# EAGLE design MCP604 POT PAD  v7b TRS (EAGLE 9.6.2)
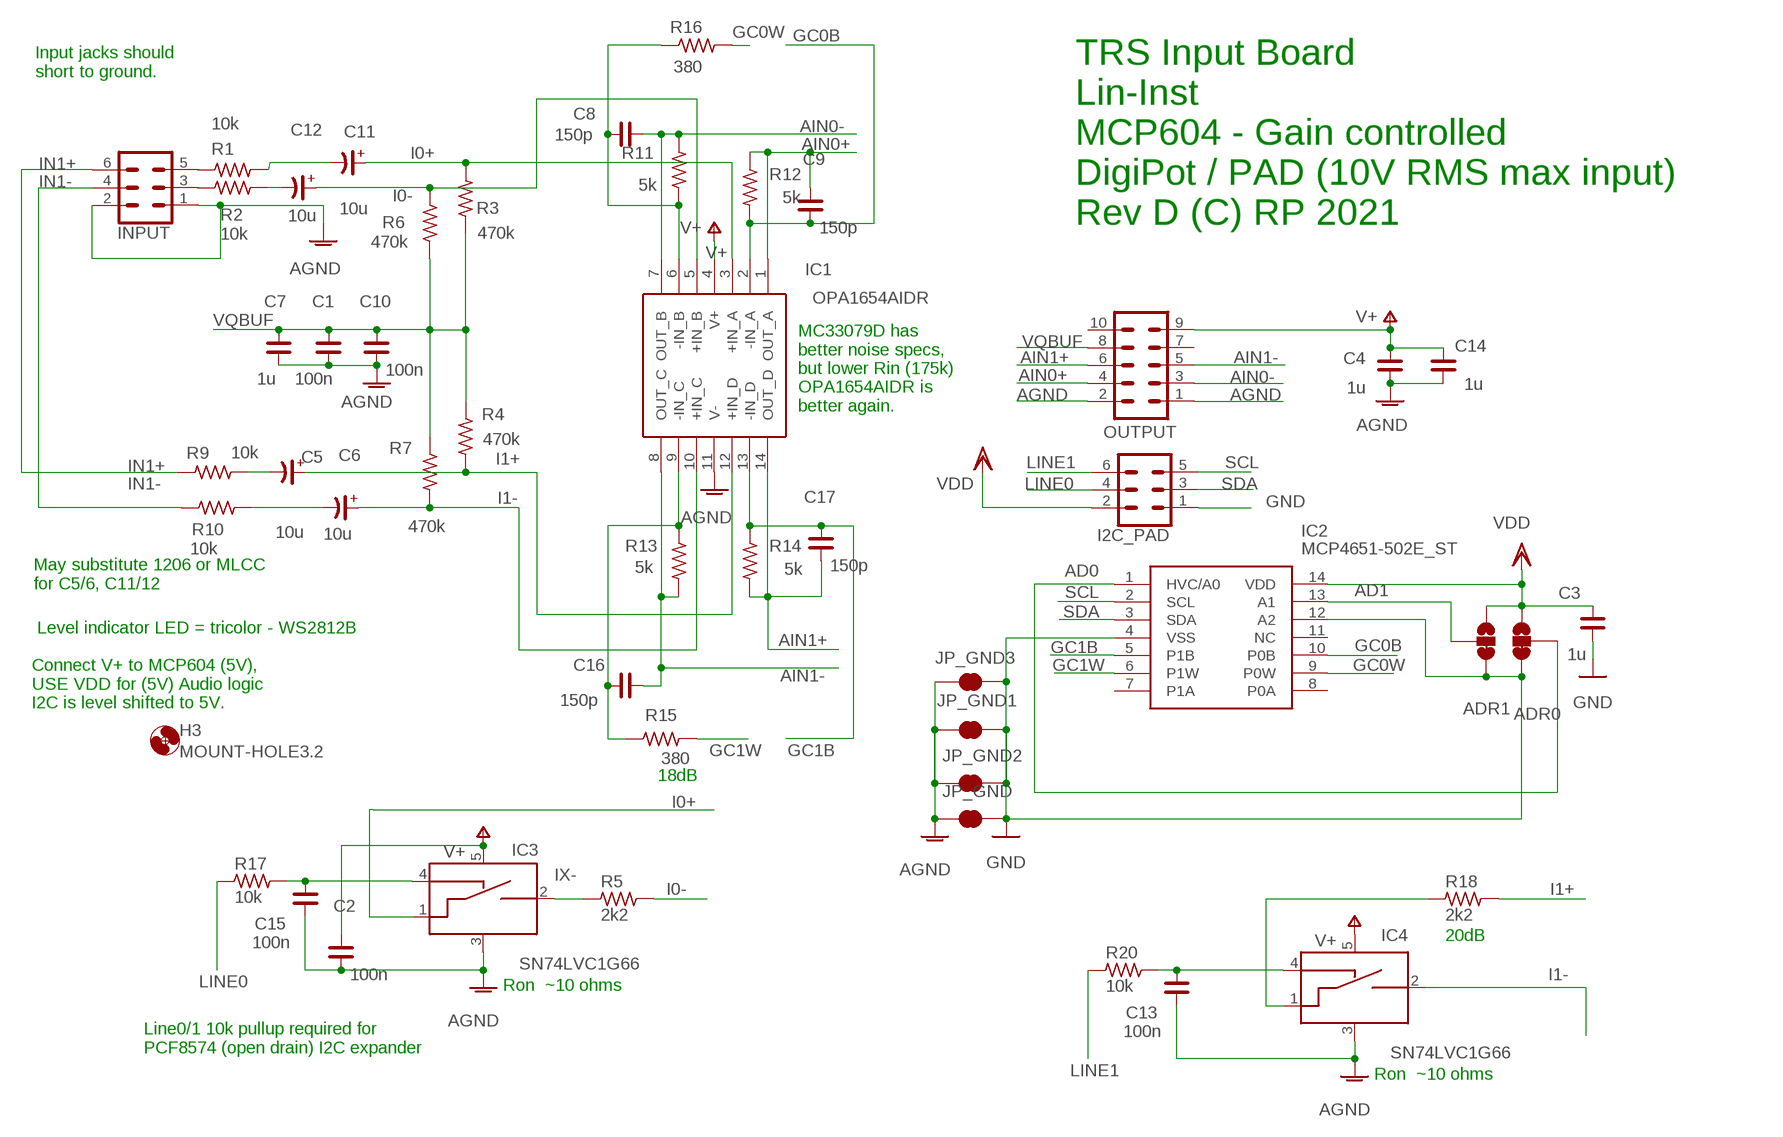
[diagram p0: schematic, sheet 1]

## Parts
ADR0  JUMPER-SMT_3_1-NC_TRACE_SILK  [SMT-JUMPER_3_1-NC_TRACE_SILK]
ADR1  JUMPER-SMT_3_1-NC_TRACE_SILK  [SMT-JUMPER_3_1-NC_TRACE_SILK]
C1  100n  C_0805  [C0805]
C2  100n  C_0805  [C0805]
C3  1u  C_0805  [C0805]
C4  1u  C_0805  [C0805]
C5  10u  CP_SV-B  [CSV-B]
C6  10u  CP_SV-B  [CSV-B]
C7  1u  C_0805  [C0805]
C8  150p  C_0805  [C0805]
C9  150p  C_0805  [C0805]
C10  100n  C_0805  [C0805]
C11  10u  CP_SV-B  [CSV-B]
C12  10u  CP_SV-B  [CSV-B]
C13  100n  C_0805  [C0805]
C14  1u  C_0805  [C0805]
C15  100n  C_0805  [C0805]
C16  150p  C_0805  [C0805]
C17  150p  C_0805  [C0805]
H3  MOUNT-HOLE3.2  [3,2]
I2C_PAD  CONN_03X2SHROUD  [2X3-SHROUDED]
IC1  OPA1654AIDR  [SOIC127P600X175-14N]
IC2  MCP4651-502E_ST  [SOP65P640X120-14N]
IC3  SN74LVC1G66  74LVC1G66  [SOT23-5]
IC4  SN74LVC1G66  74LVC1G66  [SOT23-5]
INPUT  CONN_03X2SHROUD  [2X3-SHROUDED]
JP_GND  JUMPER-SMT_2_NC_TRACE_NO-SILK  [SMT-JUMPER_2_NC_TRACE_NO-SILK]
JP_GND1  JUMPER-SMT_2_NC_TRACE_NO-SILK  [SMT-JUMPER_2_NC_TRACE_NO-SILK]
JP_GND2  JUMPER-SMT_2_NC_TRACE_NO-SILK  [SMT-JUMPER_2_NC_TRACE_NO-SILK]
JP_GND3  JUMPER-SMT_2_NC_TRACE_NO-SILK  [SMT-JUMPER_2_NC_TRACE_NO-SILK]
OUTPUT  CONN_05X2SHD_LOCK  [2X5-SHROUDED_LOCK]
R1  10k  R_0805  [R0805]
R2  10k  R_0805  [R0805]
R3  470k  R_0805  [R0805]
R4  470k  R_0805  [R0805]
R5  2k2  R_0805  [R0805]
R6  470k  R_0805  [R0805]
R7  470k  R_0805  [R0805]
R9  10k  R_0805  [R0805]
R10  10k  R_0805  [R0805]
R11  5k  R_0805  [R0805]
R12  5k  R_0805  [R0805]
R13  5k  R_0805  [R0805]
R14  5k  R_0805  [R0805]
R15  380  R_0805  [R0805]
R16  380  R_0805  [R0805]
R17  10k  R_0805  [R0805]
R18  2k2  R_0805  [R0805]
R20  10k  R_0805  [R0805]

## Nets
AD0: ADR0.2 IC2.1(HVC/A0)
AD1: ADR1.2 IC2.13(A1)
AGND: C1.1 C2.1 C4.1 C7.1 C10.1 C13.1 C14.1 C15.1 IC1.11(V-) IC3.3(VSS) IC4.3(VSS) INPUT.1 INPUT.2 JP_GND1.1 JP_GND2.1 JP_GND3.1 JP_GND.1 OUTPUT.1 OUTPUT.2
AIN0+: C9.2 IC1.1(OUT_A) OUTPUT.4 R12.2
AIN0-: C8.1 IC1.7(OUT_B) OUTPUT.3 R11.2
AIN1+: C17.1 IC1.14(OUT_D) OUTPUT.6 R14.1
AIN1-: C16.1 IC1.8(OUT_C) OUTPUT.5 R13.1
GC0B: C9.1 IC1.2(-IN_A) IC2.10(P0B) R12.1
GC0W: IC2.9(P0W) R16.1
GC1B: C17.2 IC1.13(-IN_D) IC2.5(P1B) R14.2
GC1W: IC2.6(P1W) R15.1
GND: ADR0.3 ADR1.3 C3.1 I2C_PAD.1 IC2.4(VSS) IC2.12(A2) JP_GND1.2 JP_GND2.2 JP_GND3.2 JP_GND.2
I0+: C11.+ IC1.3(+IN_A) IC3.1(A_IN) R3.2
I0-: C12.+ IC1.5(+IN_B) R5.2 R6.2
I1+: C5.+ IC1.12(+IN_D) R4.1 R18.2
I1+X: IC4.1(A_IN) R18.1
I1-: C6.+ IC1.10(+IN_C) IC4.2(A_OUT) R7.1
IN1+: INPUT.6 R9.1
IN1-: INPUT.4 R10.1
IX-: IC3.2(A_OUT) R5.1
LINE0: I2C_PAD.4 R17.1
LINE1: I2C_PAD.6 R20.1
N$2: C12.- R2.2
N$4: C13.2 IC4.4(CTRL_IN) R20.2
N$5: C8.2 IC1.6(-IN_B) R11.1 R16.2
N$6: INPUT.5 R1.1
N$7: C16.2 IC1.9(-IN_C) R13.2 R15.2
N$8: INPUT.3 R2.1
N$9: C11.- R1.2
N$15: C15.2 IC3.4(CTRL_IN) R17.2
N$18: C5.- R9.2
N$19: C6.- R10.2
SCL: I2C_PAD.5 IC2.2(SCL)
SDA: I2C_PAD.3 IC2.3(SDA)
V+: C2.2 C4.2 C14.2 IC1.4(V+) IC3.5(VCC) IC4.5(VCC) OUTPUT.9
VDD: ADR0.1 ADR1.1 C3.2 I2C_PAD.2 IC2.14(VDD)
VQBUF: C1.2 C7.2 C10.2 OUTPUT.8 R3.1 R4.2 R6.1 R7.2
Unconnected: IC2.7(P1A) IC2.8(P0A) IC2.11(NC) OUTPUT.7 OUTPUT.10

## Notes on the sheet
- Input jacks should 
  short to ground.
- TRS Input Board
  Lin-Inst
  MCP604 - Gain controlled
  DigiPot / PAD (10V RMS max input)
  Rev D (C) RP 2021
- MC33079D has
  better noise specs,
  but lower Rin (175k)
  OPA1654AIDR is 
  better again.
- May substitute 1206 or MLCC 
  for C5/6, C11/12
- Level indicator LED = tricolor - WS2812B
- Connect V+ to MCP604 (5V), 
  USE VDD for (5V) Audio logic
  I2C is level shifted to 5V.
- 18dB
- 20dB
- Ron  ~10 ohms
- Line0/1 10k pullup required for 
  PCF8574 (open drain) I2C expander
- Ron  ~10 ohms

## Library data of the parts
ADR0 ADR1 = MY-SparkFun-Jumpers:JUMPER-SMT_3_1-NC_TRACE: Normally closed trace jumper (1 of 2 connections) This jumper has a trace between two pads so it's normally closed (NC). The other connection is normally open (NO). Use a razor knife to open the connection. For best results follow the IPC guidelines for cutting traces: Cutout at least 0.063 mm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
C1-C4 C7-C10 C13-C17 = rc-master-smd:C_: NON-POLARIZED CAP
C5 C6 C11 C12 = rc-master-smd:CP_: POLARIZED CAP
H3 = holes:MOUNT-HOLE: MOUNTING HOLE with drill center marker
I2C_PAD INPUT = SparkFun-Connectors:CONN_03X2: Multi connection point. Often used as Generic Header-pin footprint for 0.1 inch spaced/style header connections You can populate with any combo of single row headers, but if you'd like an exact match, check these: Header - 2x3 (Male, 0.1") (PRT-12807) Header - 2x3 (Female, 0.1") (PRT-13010) 2x3 Pin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; PROD_ID: CONN-10681; SF_ID: PRT_10877
IC1 = SamacSys_Parts:OPA1654AIDR: Quad sound plus low noise and distortion, general-purpose, FET-input audio op amps Source: Datasheet; DESCRIPTION: Quad sound plus low noise and distortion, general-purpose, FET-input audio op amps; HEIGHT: 1.75mm; MANUFACTURER_NAME: Texas Instruments; MANUFACTURER_PART_NUMBER: OPA1654AIDR; MOUSER_PART_NUMBER: 595-OPA1654AIDR; MOUSER_PRICE-STOCK: https://www.mouser.co.uk/ProductDetail/Texas-Instruments/OPA1654AIDR/?qs=3jfYfyvUSwBoAaznhYMhNg%3D%3D
IC2 = SamacSys_Parts:MCP4651-502E_ST: Digital Potentiometer 256 Step 5kOhm Source: Datasheet; DESCRIPTION: Digital Potentiometer 256 Step 5kOhm; HEIGHT: 1.2mm; MANUFACTURER_NAME: Microchip; MANUFACTURER_PART_NUMBER: MCP4651-502E/ST; MOUSER_PART_NUMBER: 579-MCP4651-502E/ST; MOUSER_PRICE-STOCK: https://www.mouser.co.uk/ProductDetail/Microchip-Technology/MCP4651-502E-ST/?qs=hH%252BOa0VZEiDW0L9aQHIQAA%3D%3D
IC3 IC4 = SparkFun-IC-Logic:74*1G66: SN74LVC1G66 - SPST NO Analog Switch Specifications: 10-Ohm on resistance 1.65-5.5V TI Datasheet Example device(s): Spectacle; PROD_ID: IC-13549
JP_GND JP_GND1-JP_GND3 = MY-SparkFun-Jumpers:JUMPER-SMT_2_NC_TRACE: Normally closed trace jumper
OUTPUT = SparkFun-Connectors:CONN_05X2: Multi connection point. Often used as Generic Header-pin footprint for 0.1 inch spaced/style header connections For AVR SPI programming port, see special device with nice symbol: "AVR_SPI_PROG_5x2.dev" You can populate with any combo of single row headers, but if you'd like an exact match, check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; PROD_ID: CONN-08671; SF_ID: PRT-08506
R1-R7 R9-R18 R20 = rc-master-smd:R_: RESISTOR

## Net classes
0 default: width 0.152 mm
3 power: width 0.305 mm

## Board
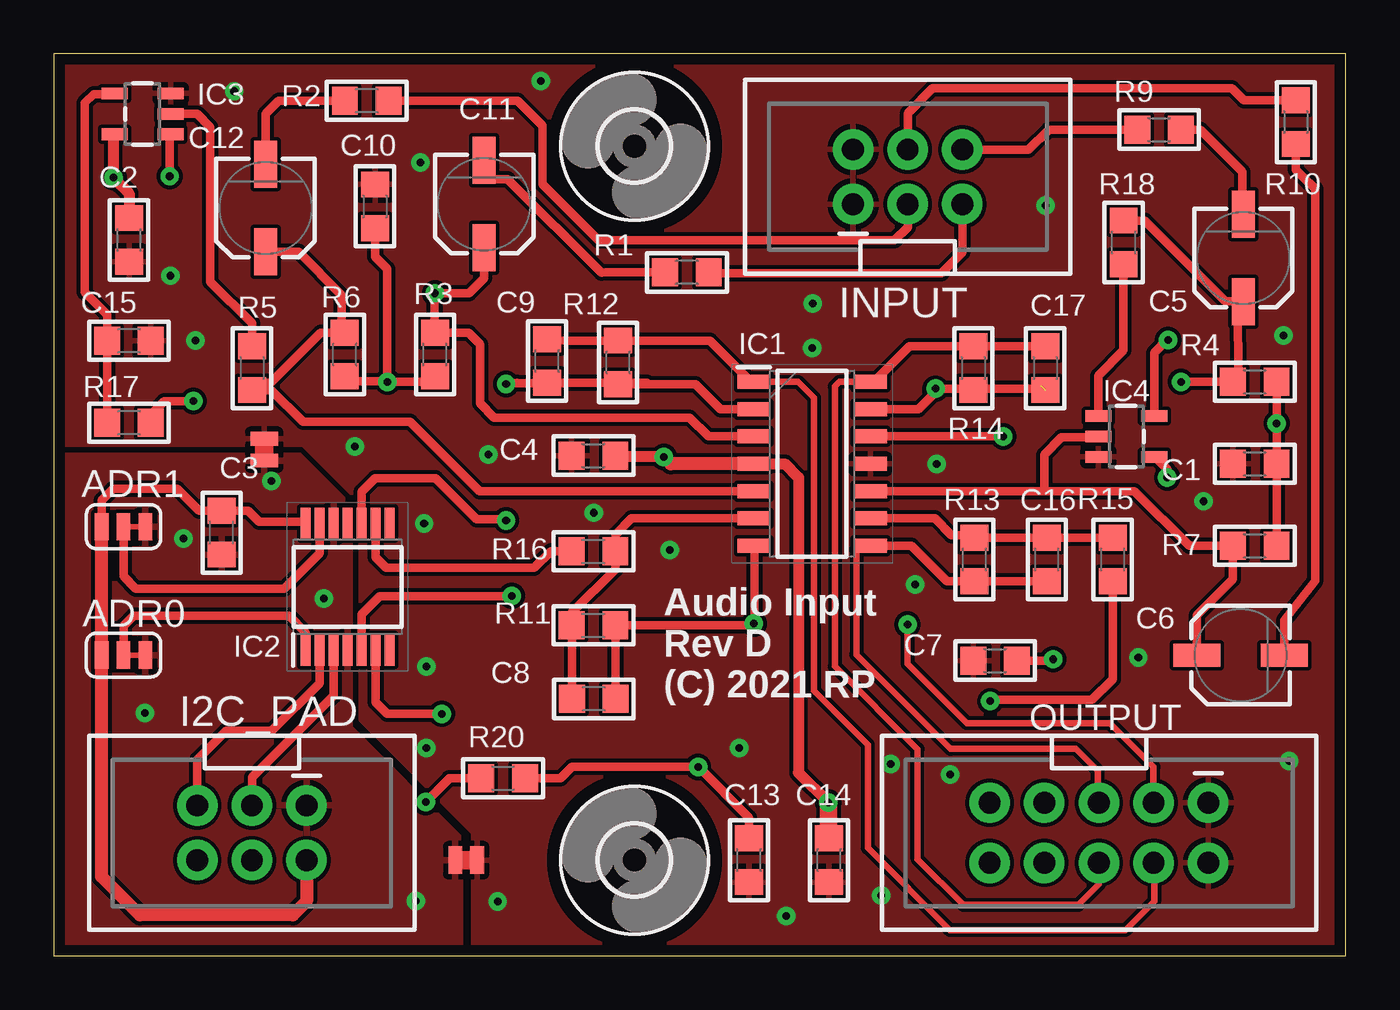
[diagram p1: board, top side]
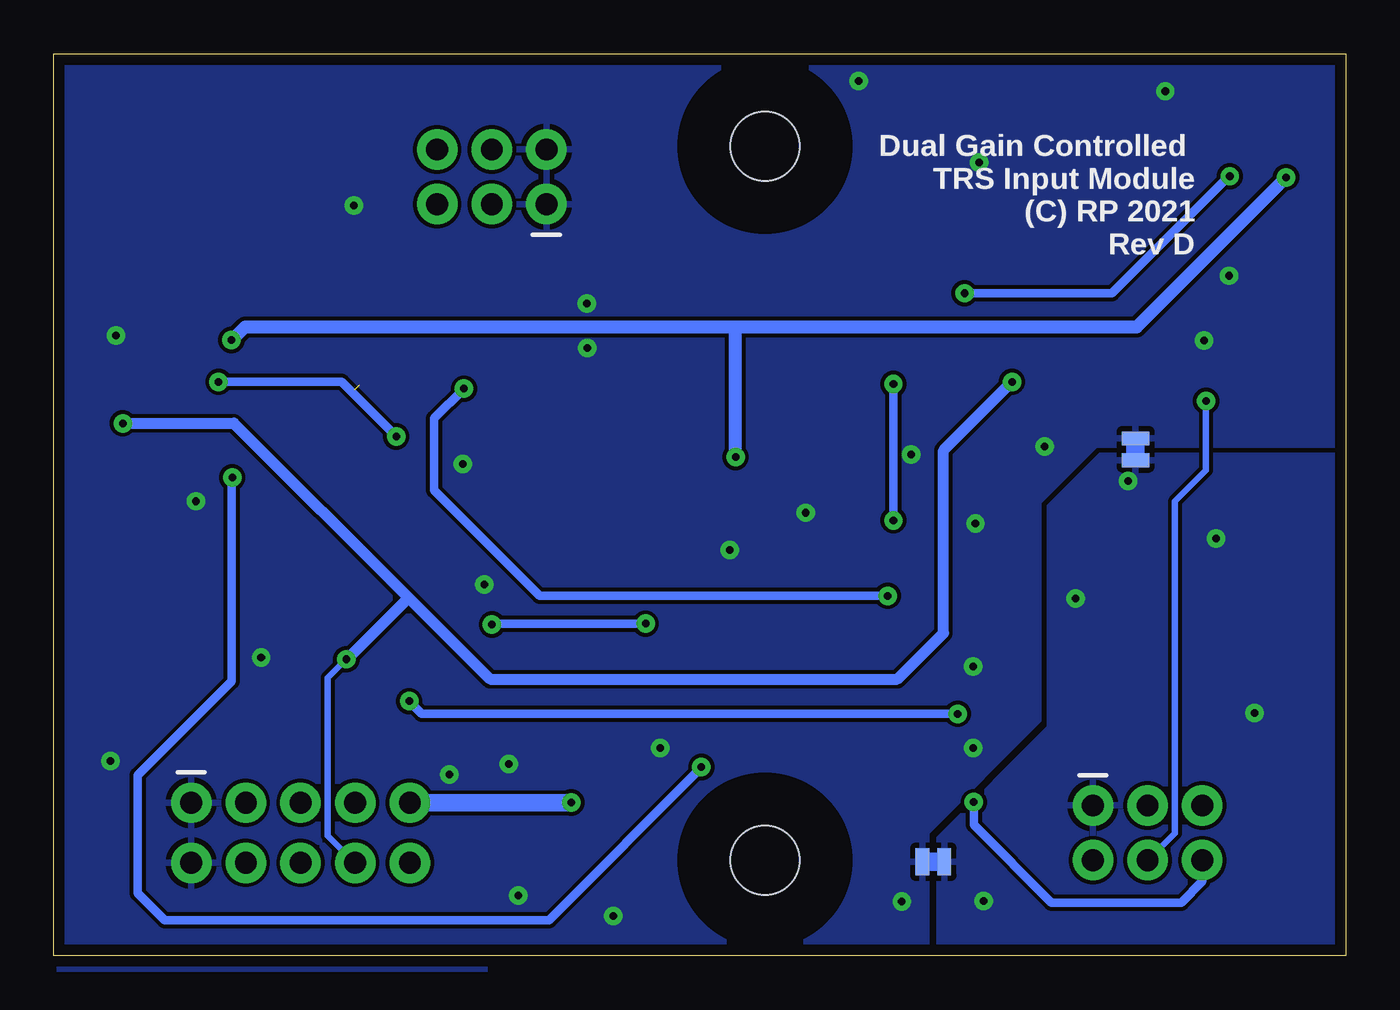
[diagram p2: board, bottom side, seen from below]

Size 60.05 x 41.91 mm. Coordinates in mm from the lower left corner, seen from the top.
Outline: 60.05,41.91 0,41.91 0,0 60.05,0 60.05,41.91
Copper layers (1*16): Top 0.035mm / dielectric 1.5mm / Bottom 0.035mm
Design rules "SparkFun - PCBWAY": minimum track width 8mil, minimum drill 13.5mil, track to track 7mil, track to pad 7mil, pad to pad 7mil, via to via 7mil, smd to smd 8mil, copper to edge 20mil, drill to drill 8mil, minimum pad ring 12mil, minimum via ring 10mil, stop-mask expansion 4mil, vias tented up to drill 25mil, thermal gap 10mil

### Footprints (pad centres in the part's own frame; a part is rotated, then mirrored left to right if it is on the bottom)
SMT-JUMPER_3_1-NC_TRACE_SILK = smd 0.635 x 1.27: 1 -1.016,0; 2 0,0; 3 1.016,0
C0805 = smd 1.2 x 1.3: 1 -1.016,0; 2 1.016,0
CSV-B = smd 2.184 x 1.067: + -2.032,0; - 2.032,0
3,2 = hole 3.2: 0,0
2X3-SHROUDED = drill 1.016 pad 1.88: 1 -1.27,2.54; 2 1.27,2.54; 3 -1.27,0; 4 1.27,0; 5 -1.27,-2.54; 6 1.27,-2.54
SOIC127P600X175-14N = smd 1.525 x 0.65: 1 -2.712,3.81; 2 -2.712,2.54; 3 -2.712,1.27; 4 -2.712,0; 5 -2.712,-1.27; 6 -2.712,-2.54; 7 -2.712,-3.81; 8 2.712,-3.81; 9 2.712,-2.54; 10 2.712,-1.27; 11 2.712,0; 12 2.712,1.27; 13 2.712,2.54; 14 2.712,3.81
SOP65P640X120-14N = smd 1.475 x 0.45: 1 -2.938,1.95; 2 -2.938,1.3; 3 -2.938,0.65; 4 -2.938,0; 5 -2.938,-0.65; 6 -2.938,-1.3; 7 -2.938,-1.95; 8 2.938,-1.95; 9 2.938,-1.3; 10 2.938,-0.65; 11 2.938,0; 12 2.938,0.65; 13 2.938,1.3; 14 2.938,1.95
SOT23-5 = smd 0.55 x 1.2: 1 -0.95,-1.3; 2 0,-1.3; 3 0.95,-1.3; 4 0.95,1.3; 5 -0.95,1.3
SMT-JUMPER_2_NC_TRACE_NO-SILK = smd 0.635 x 1.27: 1 -0.508,0; 2 0.508,0
2X5-SHROUDED_LOCK = drill 1.016 pad 1.88: 1 -1.397,5.08; 2 1.397,5.08; 3 -1.397,2.54; 4 1.397,2.54; 5 -1.397,0; 6 1.397,0; 7 -1.397,-2.54; 8 1.397,-2.54; 9 -1.397,-5.08; 10 1.397,-5.08
R0805 = smd 1.2 x 1.3: 1 -1.016,0; 2 1.016,0

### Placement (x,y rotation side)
ADR0  3.24,13.97 0 top
ADR1  3.24,19.94 0 top
C1  55.82,22.86 0 top
C2  3.49,33.26 90 top
C3  7.8,19.66 90 top
C4  25.09,23.24 0 top
C5  55.29,32.42 90 top
C6  55.16,13.97 0 top
C7  43.75,13.72 0 top
C8  25.1,11.94 180 top
C9  22.93,27.64 90 top
C10  14.93,34.82 270 top
C11  20,34.92 90 top
C12  9.85,34.75 90 top
C13  32.31,4.45 90 top
C14  36.03,4.45 90 top
C15  3.49,28.57 180 top
C16  46.15,18.41 90 top
C17  46.08,27.3 270 top
H1  MOUNT-HOLE3.2  [3,2]  26.99,37.62 270 top
H3  26.99,4.45 270 top
I2C_PAD  9.21,5.71 270 top
IC1  35.24,22.86 0 top
IC2  13.66,17.14 90 top
IC3  4.13,39.12 90 top
IC4  49.85,24.13 270 top
INPUT  39.69,36.2 90 top
JP_GND  19.17,4.45 180 top
JP_GND1  19.17,4.37 0 bottom
JP_GND2  9.78,23.52 270 top
JP_GND3  9.77,23.53 270 bottom
OUTPUT  48.58,5.71 270 top
R1  29.43,31.75 180 top
R2  14.54,39.73 180 top
R3  17.72,27.94 90 top
R4  55.82,26.67 0 top
R5  9.21,27.3 270 top
R6  13.53,27.94 90 top
R7  55.82,19.05 0 top
R9  51.37,38.39 0 top
R10  57.72,38.73 270 top
R11  25.09,15.35 0 top
R12  26.23,27.57 90 top
R13  42.79,18.41 90 top
R14  42.74,27.3 270 top
R15  49.22,18.41 90 top
R16  25.09,18.8 0 top
R17  3.49,24.77 180 top
R18  49.72,33.15 90 top
R20  20.88,8.26 0 top

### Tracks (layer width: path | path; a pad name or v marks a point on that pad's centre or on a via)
AD0
  Top 0.406: ADR0.2 3.24,15.33 3.7,15.79 10.93,15.79 11.71,15.02 IC2.1
AD1
  Top 0.406: ADR1.2 3.24,17.63 3.81,17.06 10.71,17.06 12.36,18.7 IC2.13
AGND  (via drill 0.35)
  other vias: 41.04,22.85 20.2,23.29 8.38,40.17 57.17,28.82 6.58,28.59 28.63,18.86 17.03,36.87 40.05,17.25 38.46,2.81 35.26,28.23 38.9,8.92 20.63,2.53 25.1,20.59 22.63,40.64 31.87,9.65 5.41,31.6 50.41,13.87 46.09,34.86 41.66,8.43 53.44,21.12 34.05,1.84 17.21,20.09 57.42,9.06 35.28,30.31 13.99,23.67 17.33,9.66 17.33,13.44
  pour Bottom: 60.28,42.3 -0.21,42.3 -0.21,23.74 11.62,23.74 14.28,21.08 14.28,10.95 19.5,5.73 19.5,-0.58 60.28,-0.63
  pour Top: 60.28,42.3 -0.21,42.3 -0.21,23.74 11.6,23.74 14.26,21.07 14.26,10.96 19.5,5.73 19.5,-0.56 60.28,-0.6
AIN0+
  Top 0.305: IC1.1 34.59,26.67 35.33,25.92 35.33,12.32 37.84,9.82 37.84,5.02 41.66,1.19 49.8,1.19 51.15,2.54 51.15,4.29 OUTPUT.4
  Top 0.406: IC1.1 32.41,26.67 30.49,28.59 R12.2 23.88,28.59 C9.2
AIN0-  (via drill 0.35)
  Top 0.305: v39.68,15.39 39.68,13.56 42.43,10.81 49.08,10.81 51.11,8.78 51.11,7.12 OUTPUT.3
  Top 0.406: IC1.7 32.56,19.01 32.58,15.47 v32.54,15.43 32.54,15.35 R11.2 26.1,12.27 C8.1
  Bottom 0.406: v39.68,15.39 39.64,15.43 v32.54,15.43
AIN1+
  Top 0.305: IC1.14 36.52,26.67 36.3,26.45 36.3,13.45 40.15,9.6 40.15,4.5 42.28,2.36 47.62,2.36 48.58,3.33 OUTPUT.6
  Top 0.406: IC1.14 38.12,26.67 39.77,28.32 R14.1 C17.1
AIN1-
  Top 0.305: IC1.8 37.46,19.05 37.3,18.89 37.3,13.99 41.68,9.61 47.5,9.61 48.52,8.6 48.52,7.17 OUTPUT.5
  Top 0.406: IC1.8 39.87,19.05 41.51,17.41 42.79,17.41 R13.1 C16.1
GC0B  (via drill 0.35)
  Top 0.406: 21.54,26.62 v21.02,26.57 21.53,26.61 23.8,26.61 C9.1 27.56,26.62 R12.1 27.63,26.56 29.82,26.56 30.98,25.4 IC1.2 | IC2.10 14.3,21.57 14.93,22.19 17.74,22.19 19.65,20.28 20.97,20.28 v21.02,20.23
  Bottom 0.406: v21.02,26.57 | v21.02,26.57 v21.02,20.23
GC0W
  Top 0.406: R16.1 23.1,18.8 22.33,18.02 15.46,18.02 14.96,18.52 IC2.9
GC1B  (via drill 0.35)  (1 unrouted)
  Top 0.406: R14.2 42.67,26.35 41.15,26.35 | 41.15,26.35 40.2,25.4 IC1.13 | 41.15,26.35 v40.98,26.35 45.68,26.35 45.85,26.52 | v21.29,16.73 21.26,16.7 15.13,16.7 14.3,15.87 IC2.5
  Bottom 0.406: v40.98,26.35 42.37,24.97 42.37,21.63 37.47,16.73 v21.29,16.73
GC1W  (via drill 0.35)
  Top 0.406: R15.1 49.22,12.85 48.25,11.89 43.58,11.89 v43.52,11.84 | IC2.6 14.95,14.21 14.95,11.79 15.5,11.24 v18.04,11.24
  Bottom 0.406: v18.04,11.24 18.04,11.25 42.94,11.25 v43.52,11.84
GND  (via drill 0.35)
  other vias: 12.55,16.61 6.02,19.38 16.83,2.54 4.24,11.29 10.11,22.06
  pour Bottom: -0.25,23.23 11.39,23.23 13.74,20.88 13.74,10.62 18.89,5.47 18.89,-0.51 -0.25,-0.51
  pour Top: -0.25,23.23 11.43,23.23 13.74,20.92 13.74,10.62 18.89,5.47 18.89,-1.07 -0.25,-1.07
I0+  (via drill 0.35)
  Top 0.406: IC1.3 30.43,24.13 29.55,25.01 20.47,25.01 19.81,25.67 19.81,28.41 19.27,28.96 R3.2 17.71,28.97 17.71,30.73 v17.72,30.79 19.31,30.79 20,31.48 C11.+ | IC3.1 5.39,38.12 v5.39,36.22
  Bottom 0.406: v17.72,30.79 10.86,30.79 5.41,36.24 v5.39,36.22
I0-
  Top 0.406: IC1.5 19.79,21.59 16.56,24.82 11.59,24.82 10.11,26.29 R5.2 9.02,26.63 10.07,26.63 12.4,28.96 R6.2 13.39,28.88 13.39,30.7 11.37,32.72 C12.+
I1+  (via drill 0.35)
  Top 0.406: R18.2 50.7,34.16 54.45,30.42 55.26,30.42 C5.+ 55.03,30.14 55.06,26.92 R4.1 v52.39,26.67 | IC1.12 v44.13,24.13
  Bottom 0.406: v44.13,24.13 46.67,26.67 v52.39,26.67
I1+X
  Top 0.406: R18.1 49.72,28.13 48.55,26.96 IC4.1
I1-
  Top 0.406: C6.+ 53.13,15.82 54.8,17.5 R7.1 52.77,19.05 50.23,21.59 46.04,21.59 | 46.04,21.59 IC1.10 | IC4.2 48,24.09 46.84,24.09 46.04,23.29 46.04,21.59
IN1+
  Top 0.406: R9.1 46.24,38.39 45.3,37.45 42.24,37.45 INPUT.6
IN1-
  Top 0.406: R10.1 55.31,39.75 54.75,40.31 40.85,40.31 39.69,39.15 INPUT.4
IX-
  Top 0.406: IC3.2 6.66,39.12 7.28,38.49 7.28,31.32 9.21,29.39 R5.1
LINE0  (via drill 0.35)
  Top 0.406: R17.1 4.51,25.13 5.14,25.77 6.48,25.77 v6.49,25.78
  Bottom 0.305: I2C_PAD.4 9.2,4.45 7.94,5.7 7.94,21.12 6.49,22.57 v6.49,25.78
LINE1  (via drill 0.35)
  Top 0.406: R20.1 18.38,8.26 18.39,8.24 v17.29,7.14
  Bottom 0.406: I2C_PAD.6 6.67,3.45 7.65,2.48 13.68,2.48 17.29,6.09 v17.29,7.14
N$2
  Top 0.406: R2.2 10.46,39.73 9.85,39.12 C12.-
N$4  (via drill 0.35)
  Top 0.406: R20.2 23.56,8.26 24.08,8.78 v29.95,8.78 29.96,8.78 32.31,6.43 C13.2 | v51.76,22.23 51.76,22.6 51.17,23.18 IC4.4
  Bottom 0.406: v29.95,8.78 29.94,8.76 37.04,1.66 54.89,1.66 56.14,2.91 56.14,8.39 51.78,12.75 51.78,22.43 v51.76,22.23
N$5
  Top 0.406: IC1.6 26.86,20.32 26.1,19.56 R16.2 26.1,17.97 24.07,15.94 R11.1 24.08,15.34 C8.2
N$6
  Top 0.406: R1.1 30.46,31.71 41.25,31.71 42.23,32.69 INPUT.5
N$7
  Top 0.406: R13.2 42.67,19.55 41.72,19.55 40.95,20.32 IC1.9 | 49.14,19.36 R15.2 C16.2 R13.2 | R13.2 42.87,19.36
N$8
  Top 0.406: R2.1 21.55,39.73 22.72,38.56 22.72,35.85 25.32,33.25 39.08,33.25 39.69,33.86 INPUT.3
N$9
  Top 0.406: R1.2 25.64,31.75 25.45,31.73 21.1,36.08 20.16,36.08 20,36.23 C11.-
N$15
  Top 0.406: IC3.4 2.81,40.04 1.85,40.04 1.44,39.63 1.44,30.82 2.48,29.78 C15.2 R17.2
N$18
  Top 0.406: C5.- 55.29,34.44 55.23,34.39 55.24,36.43 53.28,38.39 R9.2
N$19
  Top 0.406: C6.- 57.19,15.58 58.63,17.42 58.63,35.65 58.36,35.92 58.33,35.92 57.72,36.52 R10.2
SCL
  Top 0.406: IC2.2 12.36,12.67 10.14,10.45 8,10.45 6.67,9.12 I2C_PAD.5
SDA
  Top 0.406: I2C_PAD.3 9.21,8.29 13.01,12.09 IC2.3
V+  (via drill 0.35)
  Top 0.406: IC4.5 51.15,28.03 51.74,28.61 v51.79,28.61
  Top 0.508: v35.99,7.12 34.61,8.51 34.62,22.22 33.98,22.86 IC1.4 | v28.37,23.18 v28.36,23.18 26.16,23.18 C4.2 | IC3.5 2.77,38.1 v2.77,36.17 2.77,36.14 3.49,35.42 C2.2
  Top 0.61: IC1.4 28.68,22.86 v28.37,23.18
  Top 0.813: v35.99,7.12 35.99,5.5 C14.2
  Bottom 0.406: 28.36,29.23 v28.36,23.18 28.37,23.19
  Bottom 0.61: v2.77,36.17 9.71,29.23 28.36,29.23 | 28.37,23.19 28.37,29.22 51.15,29.22 51.76,28.61 v51.79,28.61
  Bottom 0.813: OUTPUT.9 36.16,7.11 v35.99,7.12
VDD
  Top 0.406: ADR1.1 2.23,21.16 2.76,21.69 5.74,21.69 6.76,20.68 C3.2 9.03,20.68 9.54,20.17 11.71,20.17 IC2.14
  Top 0.61: ADR1.1 ADR0.1 2.23,3.68 4,1.91 11.12,1.91 11.75,2.54 I2C_PAD.2
VQBUF  (via drill 0.35)
  Top 0.406: v15.51,26.67 15.5,26.68 15.5,31.91 14.93,32.49 C10.2 | R6.1 13.2,26.7 15.48,26.7 v15.51,26.67 | v15.51,26.67 15.52,26.68 17.76,26.68 17.71,26.7 R3.1 | R4.2 v56.84,24.74 C1.2 R7.2 | C7.2 46.45,13.72 v46.45,13.78
  Bottom 0.305: v46.45,13.78 46.45,13.79 47.31,12.93 47.31,5.59 OUTPUT.8
  Bottom 0.406: 42.86,15.93 42.85,15.94
  Bottom 0.508: v15.51,26.67 18.7,23.48 18.7,15 20.84,12.85 39.77,12.85 42.85,15.94 | v56.84,24.74 56.82,24.75 51.68,24.75 43.56,16.64 | 43.56,16.64 42.86,15.93 | v46.45,13.78 46.43,13.77 43.56,16.64

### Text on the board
bPlace: Dual Gain Controlled / TRS Input Module / (C) RP 2021 / Rev D
tNames: Audio Input / Rev D / (C) 2021 RP

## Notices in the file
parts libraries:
SparkFun-Connectors: Licensing: Creative Commons ShareAlike 4.0 International - https://creativecommons.org/licenses/by-sa/4.0
rc-master-smd: Copyright (C) 2007, Bob Starr
